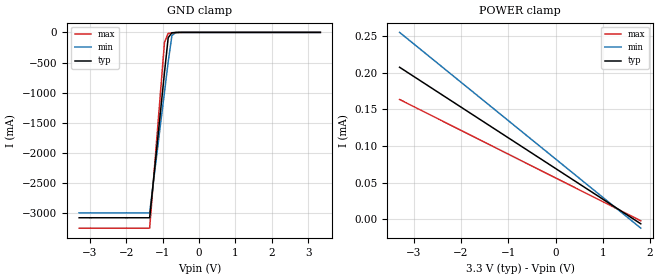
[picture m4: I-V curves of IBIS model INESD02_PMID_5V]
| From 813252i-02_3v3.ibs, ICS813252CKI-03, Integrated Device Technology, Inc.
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[Model]   INESD02_PMID_5V
Model_type   Input
Polarity   Non-Inverting
Vinl = .8V
Vinh =  2V
|   typ   min   max
C_comp   2.21pF   2.11pF   2.32pF
|   typ   min   max
[Temperature Range] 25   -40   85
[Voltage range]   3.3V   3.15V   3.45V
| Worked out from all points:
|   GND clamp passes 1 mA (typ) near -0.58 V on its own axis
[GND_clamp]
|Voltage   I(typ)   I(min)   I(max)
-3.3V     -3.072A    -2.991A    -3.244A
-1.361V   -3.072A    -2.991A    -3.244A
-952.6mV  -663.5mA   -987.5mA   -164.6mA
-850.5mV  -87.69mA   -487.6mA   -16.11mA
-748.5mV  -6.402mA   -52.83mA   -9.238mA
-646.4mV  -1.994mA   -2.763mA   -4.213mA
3.334V    70.59uA    92.59uA    52.02uA
[POWER_clamp]
|Voltage   I(typ)   I(min)   I(max)
-3.3V     207.5uA    255.1uA    163.5uA
-1.973V   151.9uA    185.6uA    120.4uA
-1.871V   147.6uA    180.2uA    117.1uA
1.803V    -6.417uA   -12.35uA   -2.293uA
